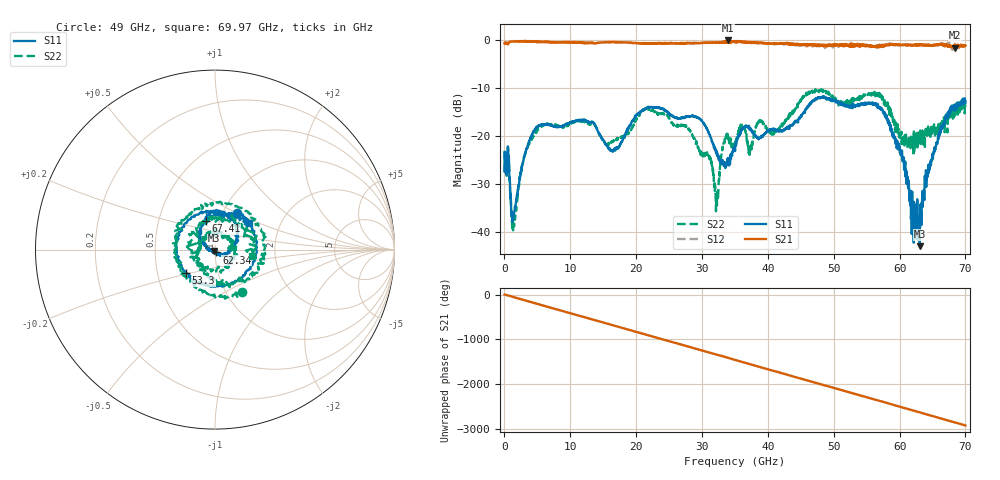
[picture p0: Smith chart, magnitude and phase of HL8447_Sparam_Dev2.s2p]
! 1/27/2023 9:38:20 AM
! D:\SMA SENSE\127\FIN\SN2.S2P
! CHANNEL.1
! TR.MEASUREMENT
! CORRECTED.DATA
# GHZ S RI R 50.0
! FREQ.GHZ  S11RE  S11IM  S21RE  S21IM  S12RE  S12IM  S22RE  S22IM
!; PortSelection: Port_12
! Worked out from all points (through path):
!   2000 points, 35 MHz to 70 GHz, reference 50 ohm
!   highest |S21| = -0.05 dB at 33.91 GHz (marker M1); lowest = -1.5 dB at 68.36 GHz (marker M2)
!   group delay of S21, straight-line fit = 116 ps
!   lowest |S11| = -43.0 dB at 63.07 GHz (marker M3), VSWR 1.01, Z = 49.6 - j0.609 ohm
!   |S11| at or under -10 dB: start of sweep to end of sweep
!   |S22| runs from -39.6 to -10.2 dB; largest |S21 - S12| = 0.1
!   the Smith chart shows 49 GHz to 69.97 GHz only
!   S11 on the Smith chart (normalised r, x): 49 GHz: 1.16, +0.51; 53.3 GHz: 0.70, -0.19; 62.34 GHz: 1.02, -0.03; 67.41 GHz: 0.86, +0.28; 69.97 GHz: 1.38, +0.43
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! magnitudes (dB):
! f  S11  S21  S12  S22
! 35 MHz  -23.3  -0.7  -0.7  -23.3
! 1.4 GHz  -36.7  -0.3  -0.2  -38.5
! 2.8 GHz  -25.7  -0.2  -0.2  -25.5
! 4.655 GHz  -18.7  -0.3  -0.3  -19.5
! 11.72 GHz  -16.7  -0.5  -0.5  -17.0
! 16.48 GHz  -23.3  -0.4  -0.4  -21.0
! 23.38 GHz  -14.0  -0.7  -0.6  -15.5
! 31.01 GHz  -19.3  -0.5  -0.5  -24.0
! 32.16 GHz  -23.4  -0.5  -0.4  -33.0
! 33.91 GHz  -24.6  0.0  -0.1  -19.6
! 35.03 GHz  -23.1  -0.4  -0.4  -21.7
! 46.69 GHz  -12.8  -1.0  -1.2  -10.6
! 49 GHz  -12.4  -1.0  -1.4  -11.0
! 53.3 GHz  -13.6  -0.9  -1.1  -12.4
! 58.34 GHz  -17.1  -1.0  -0.7  -13.5
! 62.34 GHz  -35.1  -0.9  -0.9  -20.9
! 63.07 GHz  -43.0  -0.9  -1.0  -20.9
! 64.16 GHz  -28.0  -1.0  -1.0  -19.1
! 67.41 GHz  -15.6  -1.4  -0.4  -16.4
! 68.36 GHz  -13.4  -1.5  -1.6  -14.5
! 69.97 GHz  -12.5  -1.2  -0.9  -13.5
! 70 GHz  -13.0  -1.2  -1.0  -13.9
